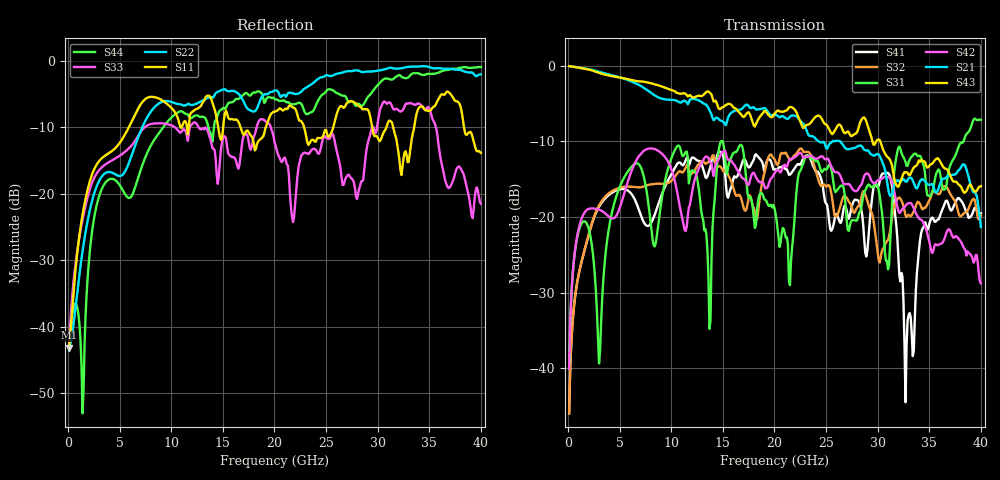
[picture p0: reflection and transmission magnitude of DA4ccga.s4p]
! ADC12DJ3200QML-SP
! 196-pin NWE package
! CCGA Ceramic Package with columns (ceramic column grid array)
! Texas Instruments 4/21/2021
! Single-ended  S-parameters
! PORT#  PORT_NAME  NET_NAME
! PORT1:  DAxN.DIEBUMP DAxN
! PORT2:  DAxN.BGA  DAxN
! PORT3:  DAxP.DIEBUMP DAxP
! PORT4:  DAxP.BGA  DAxP
! Touchstone Ver. 1.0
! Number of ports is 4
# Hz	S	MA	R	50.000000
! SCATTERING PARAMETERS  :
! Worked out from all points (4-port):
!   400 points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, 100 MHz to 40 GHz, reference 50 ohm
!   strongest paths, dB at 100 MHz, 10.1 GHz, 20.1 GHz, 30.1 GHz, 40 GHz:
!     S43: -0.1, -3.3, -6.2, -9.7, -15.9
!     S21: -0.1, -4.5, -6.5, -11.7, -21.3
!     S42: -40.0, -14.0, -14.0, -15.0, -28.7
!     S31: -40.0, -11.9, -19.6, -16.5, -7.2
!     S32: -45.9, -15.1, -12.7, -25.7, -19.8
!     S41: -45.9, -14.1, -13.7, -15.9, -19.5
!   lowest |S11| = -43.1 dB at 100 MHz (marker M1), VSWR 1.01, Z = 50.7 - j0.0531 ohm
!   |S11| at or under -10 dB: start of sweep to 5.889 GHz; 16.71 GHz to 19.16 GHz (2.446 GHz wide, 13.6 % of centre); 22.87 GHz to 25.7 GHz (2.829 GHz wide, 11.6 % of centre)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
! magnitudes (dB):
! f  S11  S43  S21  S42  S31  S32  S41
! 100 MHz  -43.1  -0.1  -0.1  -40.0  -40.0  -45.9  -45.9
! 1.4 GHz  -23.1  -0.4  -0.3  -19.9  -20.7  -25.4  -25.4
! 2.6 GHz  -16.1  -0.8  -0.6  -18.9  -27.8  -19.6  -19.8
! 7.7 GHz  -5.6  -2.2  -3.3  -11.0  -17.4  -15.8  -21.2
! 31 GHz  -9.3  -12.1  -16.1  -14.7  -26.9  -23.0  -14.2
! 32.7 GHz  -13.6  -14.1  -15.3  -18.5  -12.7  -19.8  -44.5
! 40 GHz  -13.9  -15.9  -21.3  -28.7  -7.2  -19.8  -19.5
